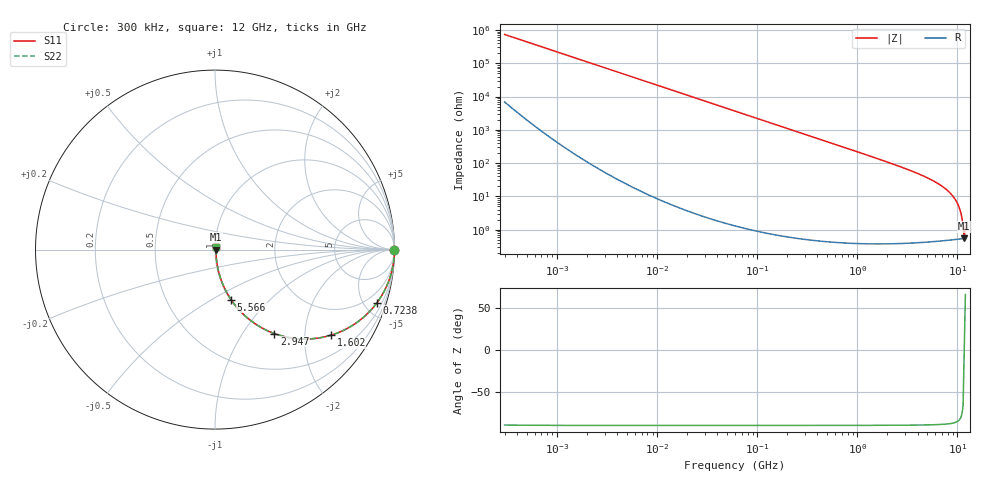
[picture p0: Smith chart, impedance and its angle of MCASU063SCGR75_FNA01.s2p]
! MCASU063SCGR75_FNA01  S-PARAMETER MODEL  ( Standard Model )
! Model Generated by TAIYO YUDEN Corporation (http://www.ty-top.com)
! Version 1.0
! TAIYO YUDEN Control No. 230609
! Copyright(c) 2023 TAIYO YUDEN CO.,LTD. All Rights Reserved.
! Product Description (link to TY-COMPAS)
! https://ds.yuden.co.jp/TYCOMPAS/or/detail?pn=MCASU063SCGR75BFNA01&u=M
! Products Name : Multilayer Ceramic Capacitors
! Characteristics :
!  Capacitance : 0.75 [pF] , Rated Voltage : 50 [V] , TCC : CG / C0G
!  Case Size : 0.6 x 0.3 / 0.024 x 0.012 [mm/inch] , Thickness : 0.3 / 0.012 [mm/inch]
!  (Conditions: Temperature = 25 [degC] , DC Bias Voltage = 0 [V])
! External Node Assignments :
!  1  o---| |---o  2
! GND o---------o GND
! Frequency Range : 0.3MHz  -  12000MHz  [ 401 STEP ]
# MHZ S RI R 50
! Freq[MHz].  S11 Real  S11 Imag  S21 Real  S21 Imag  S12 Real  S12 Imag  S22 Real  S22 Imag
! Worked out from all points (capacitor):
!   401 points, 300 kHz to 12 GHz, reference 50 ohm
!   read as one part in series: C = 722 fF near 316.3 kHz
!   lowest |Z| = 542 mohm at 11.69 GHz (marker M1)
!   series resonance near 11.68 GHz, so ESL is about 260 pH
!   S11 on the Smith chart (normalised r, x): 300 kHz: open; 723.8 MHz: 1.01, -6.07; 1.602 GHz: 1.01, -2.70; 2.947 GHz: 1.01, -1.40; 5.566 GHz: 1.01, -0.61; 12 GHz: 1.01, +0.02
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0.3  1 -0.000136  1.29e-06 0.000136  1.29e-06 0.000136  1 -0.000136
1.769972  1 -0.000802  1.52e-06 0.000802  1.52e-06 0.000802  1 -0.000802
10.44266  1 -0.00473  2.42e-05 0.00473  2.42e-05 0.00473  1 -0.00473
60  0.9993 -0.0272  0.000749 0.0272  0.000749 0.0272  0.9993 -0.0272
164.1901  0.9945 -0.074  0.00555 0.074  0.00555 0.074  0.9945 -0.074
353.9943  0.9747 -0.1566  0.0253 0.1566  0.0253 0.1566  0.9747 -0.1566
723.8279  0.9018 -0.2969  0.0982 0.2969  0.0982 0.2969  0.9018 -0.2969
1076.992  0.8044 -0.3957  0.1956 0.3957  0.1956 0.3957  0.8044 -0.3957
1602.47  0.6456 -0.477  0.3544 0.477  0.3544 0.477  0.6456 -0.477
2088.533  0.5112 -0.498  0.4888 0.498  0.4888 0.498  0.5112 -0.498
2947.191  0.3306 -0.4677  0.6694 0.4677  0.6694 0.4677  0.3306 -0.4677
4158.869  0.1793 -0.3792  0.8207 0.3792  0.8207 0.3792  0.1793 -0.3792
5565.855  0.0896 -0.2786  0.9104 0.2786  0.9104 0.2786  0.0896 -0.2786
7448.838  0.0347 -0.1702  0.9653 0.1702  0.9653 0.1702  0.0347 -0.1702
8281.503  0.0222 -0.1304  0.9778 0.1304  0.9778 0.1304  0.0222 -0.1304
9207.246  0.0133 -0.0908  0.9867 0.0908  0.9867 0.0908  0.0133 -0.0908
9708.23  0.0101 -0.071  0.9899 0.071  0.9899 0.071  0.0101 -0.071
10236.47  0.00779 -0.0513  0.9922 0.0513  0.9922 0.0513  0.00779 -0.0513
10793.46  0.00624 -0.0316  0.9938 0.0316  0.9938 0.0316  0.00624 -0.0316
11083.22  0.00576 -0.0217  0.9942 0.0217  0.9942 0.0217  0.00576 -0.0217
11686.27  0.00538 0.000216  0.9946 -0.000216  0.9946 -0.000216  0.00538 0.000216
12000  0.00559 0.0122  0.9944 -0.0122  0.9944 -0.0122  0.00559 0.0122
